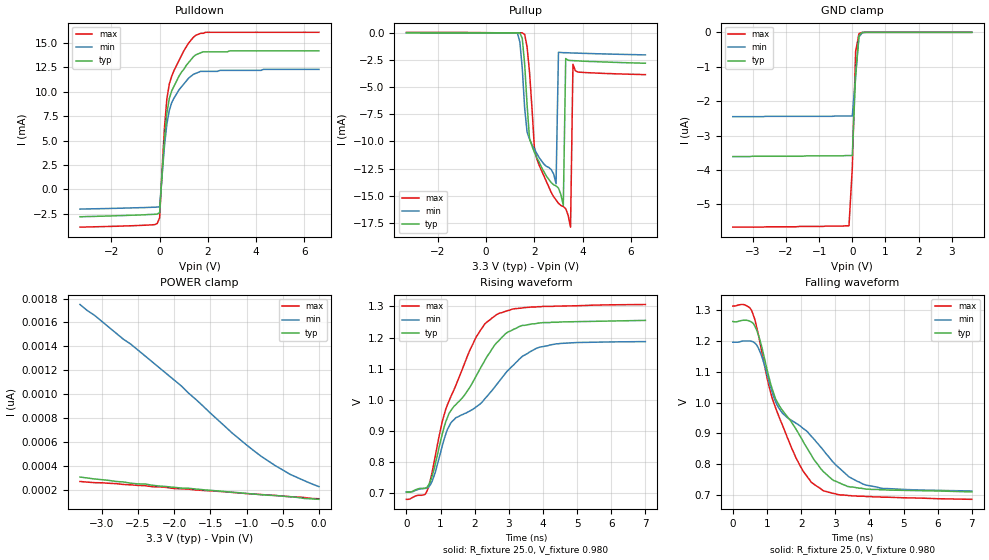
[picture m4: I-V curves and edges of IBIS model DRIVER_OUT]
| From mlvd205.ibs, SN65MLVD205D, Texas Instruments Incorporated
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|   Driver Output Model
[Model]   DRIVER_OUT
Model_type   3-state
| Signals   Y,Z
Vmeas = 1.0V   |Reference voltage for timing measurements
Cref = 3pF   |Timing specification test load capacitance value
Rref = 50   |Note: 50 Ohm load; single ended configuration
| variable   typ   min   max
C_comp   4.96pF   4.74pF   5.60pF
|   typ   min   max
[Temperature Range]   25.0   85   -40
[Voltage range]   3.3V   3.0V   3.6V
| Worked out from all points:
|   slope of the pulldown table from 0 to 0.495 V, typ, clamps not added: 39.8 ohm
|   rising waveform, R_fixture 25.0, V_fixture 0.980: 20-80 % time 1.51ns typ, 2.01ns min, 1.13ns max; typ from 0.704 V to 1.25 V
|   falling waveform, R_fixture 25.0, V_fixture 0.980: 20-80 % time 1.44ns typ, 1.93ns min, 1.09ns max; typ from 1.26 V to 0.711 V
[Pulldown]
|   Voltage   I(typ)   I(min)   I(max)
-3.3V     -2.8mA     -2.02mA    -3.87mA
-100mV    -2.53mA    -1.81mA    -3.5mA
0V        -2.37mA    -1.79mA    -2.9mA
100mV     1.53mA     1.36mA     1.99mA
200mV     5.16mA     4.45mA     6.32mA
300mV     7.82mA     6.71mA     9.29mA
400mV     9.32mA     8.09mA     10.8mA
500mV     10.1mA     8.89mA     11.6mA
800mV     11.6mA     10.2mA     13.2mA
1.4V      13.6mA     11.8mA     15.6mA
1.8V      14.1mA     12.1mA     16mA
6.6V      14.2mA     12.3mA     16.1mA
[Pullup]
|   Voltage   I(typ)   I(min)   I(max)
| Note that the[Pullup]voltage table is referenced to Vcc
| and is calculated using Vtable=Vcc - Vmeasured.
-3.3V     715nA      -518pA     46.3uA
1.3V      -10.1nA    -36.9uA    956nA
1.6V      -2.93mA    -6.97mA    -149uA
1.8V      -9.73mA    -9.79mA    -3.61mA
2V        -11mA      -10.7mA    -10.5mA
2.9V      -14.1mA    -13.9mA    -15.4mA
3V        -14.3mA    -1.79mA    -15.7mA
3.2V      -15.9mA    -1.83mA    -16mA
3.3V      -2.37mA    -1.83mA    -16.2mA
3.5V      -2.55mA    -1.85mA    -17.9mA
3.6V      -2.56mA    -1.86mA    -2.9mA
6.6V      -2.8mA     -2.03mA    -3.85mA
[GND_clamp]
|   Voltage   I(typ)   I(min)   I(max)
| Outputs in High Impedance (off)
-3.6V     -3.61uA    -2.45uA    -5.66uA
-100mV    -3.58uA    -2.43uA    -5.62uA
0V        -3.58uA    -2.43uA    -3.94uA
100mV     -1.22uA    -1.28uA    -562nA
200mV     -103nA     -135nA     -39.1nA
300mV     -3.43nA    -7.89nA    -1.42nA
400mV     -46.7pA    -554pA     -11.2pA
3.6V      140pA      404pA      129pA
[Power_clamp]
| Note that the[POWER_clamp]voltage table is referenced to Vcc
| and is calculated using Vtable=Vcc - Vmeasured.
|   Voltage   I(typ)   I(min)   I(max)
-3.3V     310pA      1.75nA     273pA
-3.2V     302pA      1.7nA      268pA
-3.1V     294pA      1.66nA     263pA
-2.7V     269pA      1.46nA     248pA
-2.6V     259pA      1.42nA     245pA
-2.4V     252pA      1.32nA     238pA
-1.9V     218pA      1.07nA     212pA
-1.2V     183pA      678pA      182pA
-900mV    168pA      530pA      168pA
-600mV    156pA      404pA      156pA
-400mV    146pA      333pA      146pA
0V        124pA      230pA      129pA
[Ramp]
|   typ   min   max
dV/dt_r   334.5mV/1.538n   294.4mV/2.069n   378.7mV/1.151n
dV/dt_f   334.2mV/1.462n   294.1mV/1.979n   378.4mV/1.103n
R_load = 25ohm  | Note: The measurement is single-ended with 25ohm
|   to ground.
[Rising Waveform]
R_fixture = 25.0
V_fixture = 0.980
V_fixture_min = 0.950
V_fixture_max = 0.997
C_fixture = 0p
L_fixture = 0n
|   V(typ)   V(min)   V(max)
0s        704mV      705mV      681mV
600ps     719mV      717mV      707mV
750ps     754mV      738mV      766mV
1.05ns    890mV      852mV      930mV
1.3ns     965mV      926mV      1.01V
2ns       1.068V     974mV      1.192V
2.35ns    1.137V     1.01V      1.249V
2.95ns    1.216V     1.092V     1.286V
3.9ns     1.247V     1.169V     1.299V
7ns       1.255V     1.187V     1.306V
[Falling Waveform]
R_fixture = 25.0
V_fixture = 0.980
V_fixture_min = 0.950
V_fixture_max = 0.997
C_fixture = 0p
L_fixture = 0n
|   V(typ)   V(min)   V(max)
0s        1.262V     1.195V     1.312V
550ps     1.26V      1.198V     1.298V
800ps     1.2V       1.163V     1.191V
1.2ns     1.029V     1.017V     999mV
1.45ns    975mV      966mV      928mV
1.85ns    914mV      933mV      821mV
2.3ns     830mV      891mV      742mV
2.95ns    748mV      806mV      706mV
3.9ns     720mV      733mV      696mV
7ns       711mV      714mV      687mV
